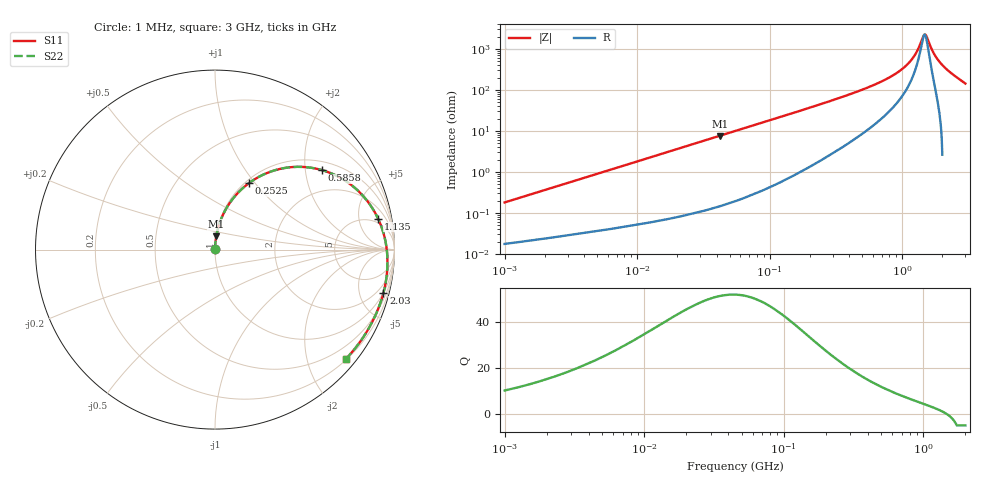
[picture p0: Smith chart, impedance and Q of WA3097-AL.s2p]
# MHz S MA R 50
!Freq  MagS11  AngS11  MagS21  AngS21  MagS12  AngS12  MagS22  AngS22
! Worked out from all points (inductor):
!   800 points, 1 MHz to 3 GHz, reference 50 ohm
!   read as one part in series: L = 28.7 nH near 1.041 MHz
!   highest Q = 52 at 42 MHz (marker M1), where L = 28.7 nH
!   self-resonance near 1.475 GHz
!   S11 on the Smith chart (normalised r, x): 1 MHz: 1.00, +0.00; 252.5 MHz: 1.04, +0.94; 585.8 MHz: 1.25, +2.47; 1.135 GHz: 3.79, +9.04; 2.03 GHz: 0.98, -7.79; 3 GHz: 0.22, -2.75
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1  0.001812 84.3  0.9998 -0.1  0.9998 -0.1  0.001812 84.3
3.83  0.00691 86.9  0.9997 -0.4  0.9997 -0.4  0.00691 86.9
14.519  0.02616 87.1  0.999 -1.5  0.999 -1.5  0.02616 87.1
41.999  0.07547 84.6  0.9957 -4.3  0.9957 -4.3  0.07547 84.6
55.047  0.09872 83.2  0.9932 -5.7  0.9932 -5.7  0.09872 83.2
120.276  0.2121 76.3  0.9718 -12.2  0.9718 -12.2  0.2121 76.3
208.704  0.3538 67.2  0.9222 -20.7  0.9222 -20.7  0.3538 67.2
252.474  0.4171 62.9  0.8908 -24.6  0.8908 -24.6  0.4171 62.9
404.346  0.5983 49.5  0.7619 -36.6  0.7619 -36.6  0.5983 49.5
585.829  0.7437 36.5  0.598 -47.7  0.598 -47.7  0.7437 36.5
791.273  0.8428 25.0  0.4281 -56.5  0.4281 -56.5  0.8428 25.0
966.859  0.8938 17.2  0.3016 -61.0  0.3016 -61.0  0.8938 17.2
1134.992  0.9247 10.8  0.1955 -62.1  0.1955 -62.1  0.9247 10.8
1254.617  0.9397 6.7  0.1284 -58.7  0.1284 -58.7  0.9397 6.7
1429.174  0.9543 1.3  0.05094 -25.6  0.05094 -25.6  0.9543 1.3
1487.621  0.9577 -0.4  0.04271 8.2  0.04271 8.2  0.9577 -0.4
1548.459  0.9607 -2.1  0.0529 41.0  0.0529 41.0  0.9607 -2.1
1677.701  0.9653 -5.6  0.1014 67.2  0.1014 67.2  0.9653 -5.6
1763.899  0.9672 -7.8  0.1377 72.3  0.1377 72.3  0.9672 -7.8
2029.549  0.9691 -14.4  0.2489 75.7  0.2489 75.7  0.9691 -14.4
2504.887  0.9634 -26.0  0.4434 72.4  0.4434 72.4  0.9634 -26.0
3000  0.9501 -39.8  0.6655 66.1  0.6655 66.1  0.9501 -39.8
